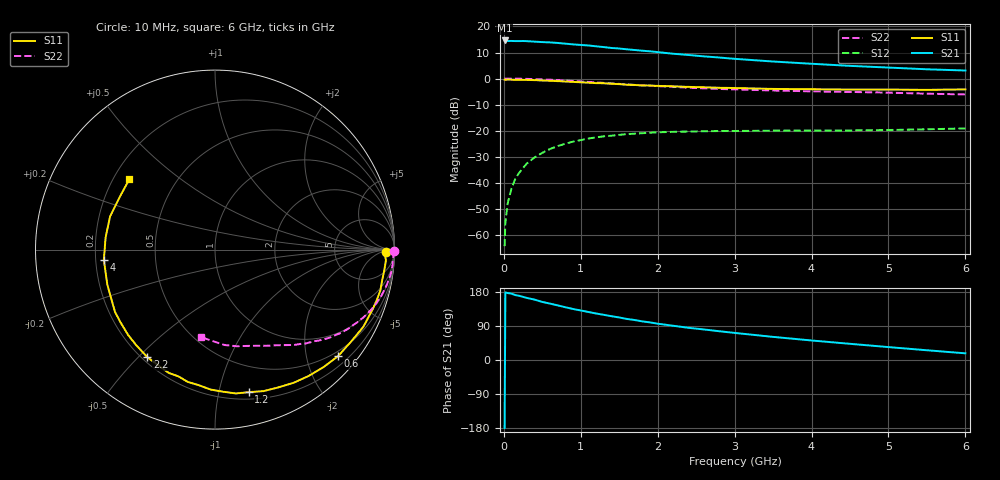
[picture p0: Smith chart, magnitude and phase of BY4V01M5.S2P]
! SIEMENS Small Signal Semiconductors
! BFY420
! Si NPN RF SIEGET Grounded Emitter Transistor in MICRO-X
! VCE = 4 V  IC = 1.5 mA
! Common Emitter S-Parameters:  October  1996
# GHz  S  MA  R  50
!  f  S11  S21  S12  S22
! GHz  MAG  ANG  MAG  ANG  MAG  ANG  MAG  ANG
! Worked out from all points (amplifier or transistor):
!   36 points, 10 MHz to 6 GHz, reference 50 ohm
!   highest |S21| = 14.6 dB at 10 MHz (marker M1)
!   |S21| within 3 dB of that: start of sweep to 1.454 GHz
!   unconditionally stable (mu >= 1): 4.233 GHz to end of sweep
!   at 250 MHz: K = 0.04, MSG = 24.4 dB, |S12| = -34.4 dB
!   at 1.4 GHz: K = 0.24, MSG = 16.9 dB, |S12| = -22.0 dB
!   at 6 GHz: K = 1.27, MAG = 8.0 dB, |S12| = -19.2 dB
!   S11 on the Smith chart (normalised r, x): 10 MHz: 37, -12; 600 MHz: 0.39, -2.63; 1.2 GHz: 0.26, -1.23; 2.2 GHz: 0.22, -0.53; 4 GHz: 0.23, -0.04; 6 GHz: 0.26, +0.34
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0.01  0.9518 -0.9  5.389 -179.6  0.0006 74.6  0.998 -0.4
0.02  0.9449 -1.4  5.364 178.6  0.0017 59.5  0.9997 -0.6
0.05  0.9542 -3.5  5.262 176.7  0.004 80.5  0.996 -1.6
0.1  0.9503 -7.1  5.274 175.0  0.0078 85.7  0.9916 -3.2
0.15  0.9469 -10.3  5.243 171.3  0.0119 81.4  0.9928 -4.8
0.2  0.9489 -13.9  5.236 169.4  0.0155 80.8  0.9912 -6.3
0.3  0.9394 -20.7  5.221 163.8  0.0234 77.2  0.984 -9.4
0.5  0.9149 -34.2  5.013 153.2  0.0373 69.6  0.9621 -15.5
0.6  0.9068 -40.9  4.942 148.9  0.0442 66.4  0.9478 -18.4
0.8  0.8762 -53.5  4.677 139.3  0.0559 58.9  0.9137 -23.9
1.1  0.8332 -71.2  4.317 126.7  0.0703 50.1  0.8593 -31.2
1.2  0.816 -76.7  4.16 122.7  0.0741 47.3  0.841 -33.5
1.6  0.7603 -97.0  3.64 108.3  0.0855 37.4  0.7701 -41.1
2  0.7219 -114.8  3.219 95.8  0.0924 30.1  0.7132 -47.3
2.2  0.7079 -122.2  2.995 90.4  0.0945 27.0  0.6914 -50.2
2.4  0.6906 -129.3  2.833 85.0  0.0957 24.5  0.6661 -53.0
2.8  0.6644 -142.4  2.533 75.9  0.098 20.2  0.6298 -57.8
3.5  0.6311 -161.8  2.123 61.0  0.0996 15.5  0.589 -65.5
4  0.6219 -174.7  1.921 51.5  0.1001 13.7  0.5669 -71.1
4.5  0.6133 173.7  1.751 42.7  0.1006 12.4  0.5525 -77.1
5.5  0.6063 151.0  1.505 25.7  0.1057 12.4  0.5115 -90.9
6  0.6179 140.6  1.425 17.6  0.1101 12.8  0.4939 -98.8
